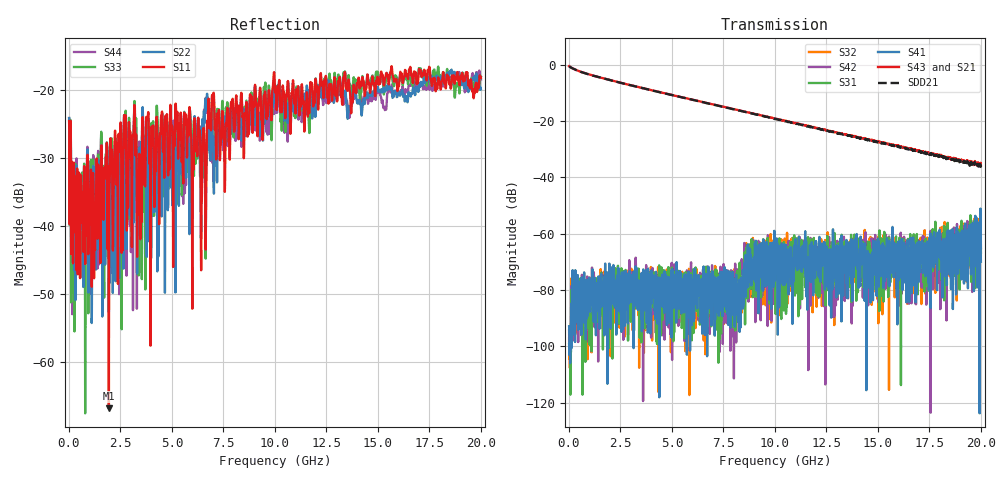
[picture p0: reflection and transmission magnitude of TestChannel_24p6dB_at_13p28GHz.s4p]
!Agilent Technologies,E5071C,MY46521579,B.13.20
!Date: Fri Mar 22 11:58:26 2024
!Data & Calibration Information:
!Freq	S11:SOLT4(ON)	S12:SOLT4(ON)	S13:SOLT4(ON)	S14:SOLT4(ON)
!	S21:SOLT4(ON)	S22:SOLT4(ON)	S23:SOLT4(ON)	S24:SOLT4(ON)
!	S31:SOLT4(ON)	S32:SOLT4(ON)	S33:SOLT4(ON)	S34:SOLT4(ON)
!	S41:SOLT4(ON)	S42:SOLT4(ON)	S43:SOLT4(ON)	S44:SOLT4(ON)
!PortZ  Port1:50+j0  Port2:50+j0  Port3:50+j0  Port4:50+j0
!Above PortZ is port z conversion or system Z0 setting when saving the data.
!When reading, reference impedance value at option line is always used.
# Hz S MA R 50
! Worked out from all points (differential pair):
!   2000 points, 10 MHz to 20 GHz, reference 50 ohm
!   strongest paths, dB at 10 MHz, 5.01 GHz, 10.01 GHz, 15.01 GHz, 20 GHz:
!     S43: -0.6, -10.8, -19.1, -27.4, -35.9
!     S21: -0.6, -10.8, -19.2, -27.5, -35.4
!     S41: -92.9, -80.7, -72.2, -72.8, -70.0
!     S31: -99.2, -83.7, -70.5, -67.5, -66.8
!     S42: -94.3, -104.9, -75.7, -76.0, -65.1
!     S32: -97.2, -72.2, -64.5, -69.8, -65.2
!   taken as a pair (ports 3,1 in; 4,2 out), SDD21 dB: -0.6, -10.8, -19.2, -27.6, -36.1
!   lowest |S11| = -66.8 dB at 1.94 GHz (marker M1), VSWR 1.00, Z = 50 + j0.0214 ohm
!   |S11| at or under -10 dB: start of sweep to end of sweep
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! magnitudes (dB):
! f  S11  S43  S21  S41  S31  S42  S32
! 10 MHz  -24.6  -0.6  -0.6  -92.9  -99.2  -94.3  -97.2
! 230 MHz  -31.6  -1.5  -1.5  -79.4  -78.4  -82.9  -78.9
! 1.94 GHz  -66.8  -5.4  -5.4  -76.8  -86.0  -74.7  -75.7
! 7.92 GHz  -22.6  -15.7  -15.7  -87.7  -91.4  -76.2  -83.0
! 8.61 GHz  -21.9  -16.8  -16.9  -68.4  -70.8  -76.7  -63.4
! 9.96 GHz  -17.4  -19.2  -19.3  -69.3  -76.3  -67.2  -73.0
! 20 GHz  -18.2  -35.9  -35.4  -70.0  -66.8  -65.1  -65.2
